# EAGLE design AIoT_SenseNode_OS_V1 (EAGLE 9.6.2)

## Sheet 1 of 4: ESP32-S3 Circuit
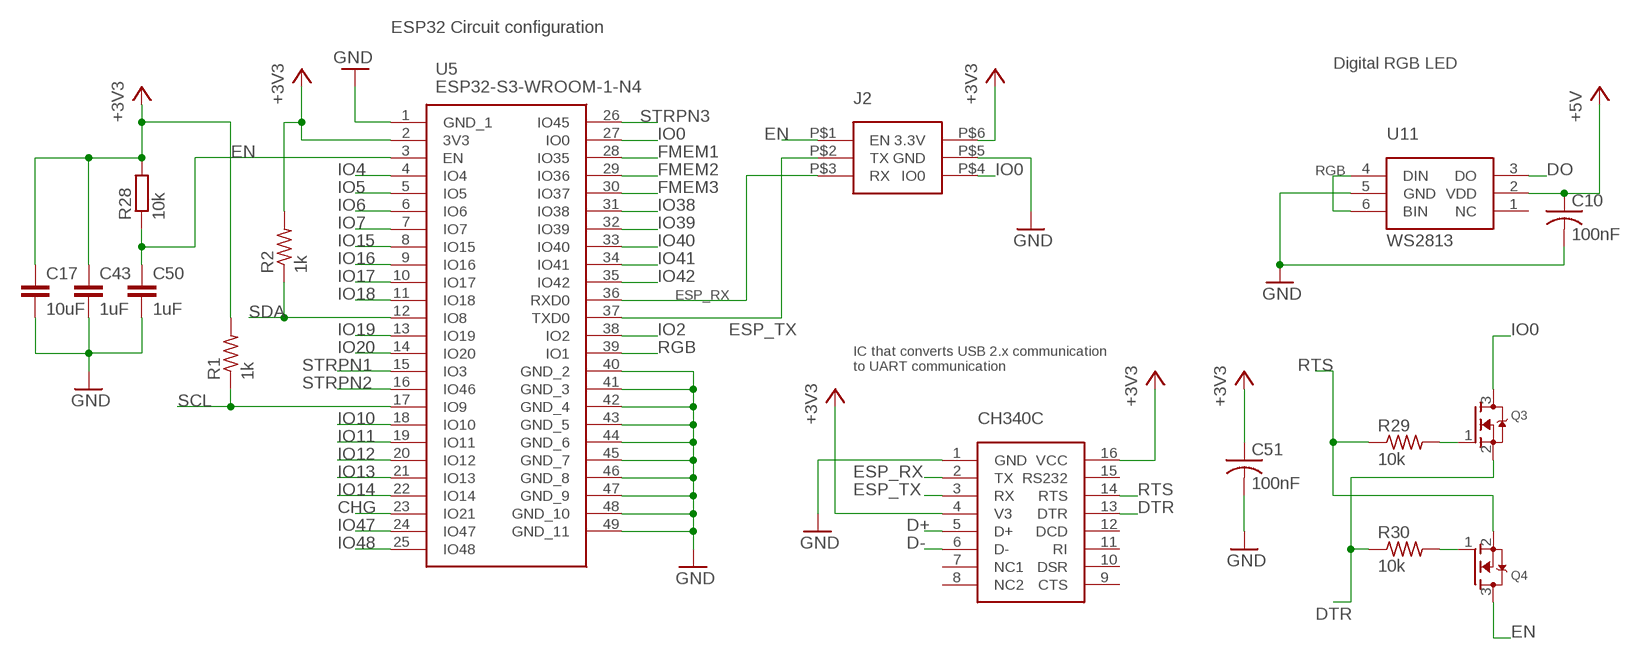
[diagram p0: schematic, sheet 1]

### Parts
C10  100nF  C-USC0603  [C0603]
C17  10uF  C-EUC0603  [C0603]
C43  1uF  C-EUC0603  [C0603]
C50  1uF  C-EUC0603  [C0603]
C51  100nF  C-USC0603  [C0603]
J2  ESP-PROG_HEADER  [2X3_1.27_HEADER]
Q3  MOSFET-NREFLOW  [SOT23-R]
Q4  MOSFET-NREFLOW  [SOT23-R]
R1  1k  R-US_R0603  [R0603]
R2  1k  R-US_R0603  [R0603]
R28  10k  R-EU_R0603  [R0603]
R29  10k  R-US_R0603  [R0603]
R30  10k  R-US_R0603  [R0603]
U5  ESP32-S3-WROOM-1-N4  [ESP32S3WROOM1N4]
U6  CH340C  [SOIC16]
U11  WS2813  [WS2813]

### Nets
+3V3: C17.1 C43.1 C51.1 J2.P$6(3.3V) R1.2 R2.2 R28.2 U5.2(3V3) U6.4(V3) U6.16(VCC) ; also sheet 2,3,4
+5V: C10.1 U11.2(VDD) ; also sheet 3
CHG: U5.23(IO21) ; also sheet 3
D+: U6.5(D+) ; also sheet 4
D-: U6.6(D-) ; also sheet 4
DO: U11.3(DO)
DTR: Q3.2(S) R30.1 U6.13(DTR)
EN: C50.1 J2.P$1(EN) Q4.3(D) R28.1 U5.3(EN) ; also sheet 4
ESP_RX: J2.P$3(RX) U5.36(RXD0) U6.2(TX)
ESP_TX: J2.P$2(TX) U5.37(TXD0) U6.3(RX)
FMEM1: U5.28(IO35)
FMEM2: U5.29(IO36)
FMEM3: U5.30(IO37)
GND: C10.2 C17.2 C43.2 C50.2 C51.2 J2.P$5(GND) U5.1(GND_1) U5.40(GND_2) U5.41(GND_3) U5.42(GND_4) U5.43(GND_5) U5.44(GND_6) U5.45(GND_7) U5.46(GND_8) U5.47(GND_9) U5.48(GND_10) U5.49(GND_11) U6.1(GND) U11.5(GND) ; also sheet 2,3,4
IO0: J2.P$4(IO0) Q3.3(D) U5.27(IO0)
IO2: U5.38(IO2) ; also sheet 4
IO4: U5.4(IO4) ; also sheet 4
IO5: U5.5(IO5) ; also sheet 4
IO6: U5.6(IO6) ; also sheet 4
IO7: U5.7(IO7) ; also sheet 4
IO10: U5.18(IO10)
IO11: U5.19(IO11) ; also sheet 4
IO12: U5.20(IO12) ; also sheet 4
IO13: U5.21(IO13) ; also sheet 4
IO14: U5.22(IO14) ; also sheet 4
IO15: U5.8(IO15) ; also sheet 4
IO16: U5.9(IO16) ; also sheet 4
IO17: U5.10(IO17) ; also sheet 4
IO18: U5.11(IO18) ; also sheet 4
IO19: U5.13(IO19) ; also sheet 4
IO20: U5.14(IO20) ; also sheet 4
IO38: U5.31(IO38) ; also sheet 4
IO39: U5.32(IO39) ; also sheet 4
IO40: U5.33(IO40) ; also sheet 4
IO41: U5.34(IO41) ; also sheet 4
IO42: U5.35(IO42) ; also sheet 4
IO47: U5.24(IO47) ; also sheet 4
IO48: U5.25(IO48) ; also sheet 4
N$3: Q4.1(G) R30.2
N$10: Q3.1(G) R29.2
RGB: U5.39(IO1) U11.4(DIN) U11.6(BIN)
RTS: Q4.2(S) R29.1 U6.14(RTS)
SCL: R1.1 U5.17(IO9) ; also sheet 2,4
SDA: R2.1 U5.12(IO8) ; also sheet 2,4
STRPN1: U5.15(IO3)
STRPN2: U5.16(IO46)
STRPN3: U5.26(IO45)
Unconnected: U6.7(NC1) U6.8(NC2) U6.9(CTS) U6.10(DSR) U6.11(RI) U6.12(DCD) U6.15(RS232) U11.1(NC)

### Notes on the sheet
- ESP32 Circuit configuration
- Digital RGB LED
- IC that converts USB 2.x communication
  to UART communication
- CH340C

## Sheet 2 of 4: ADC Circuits
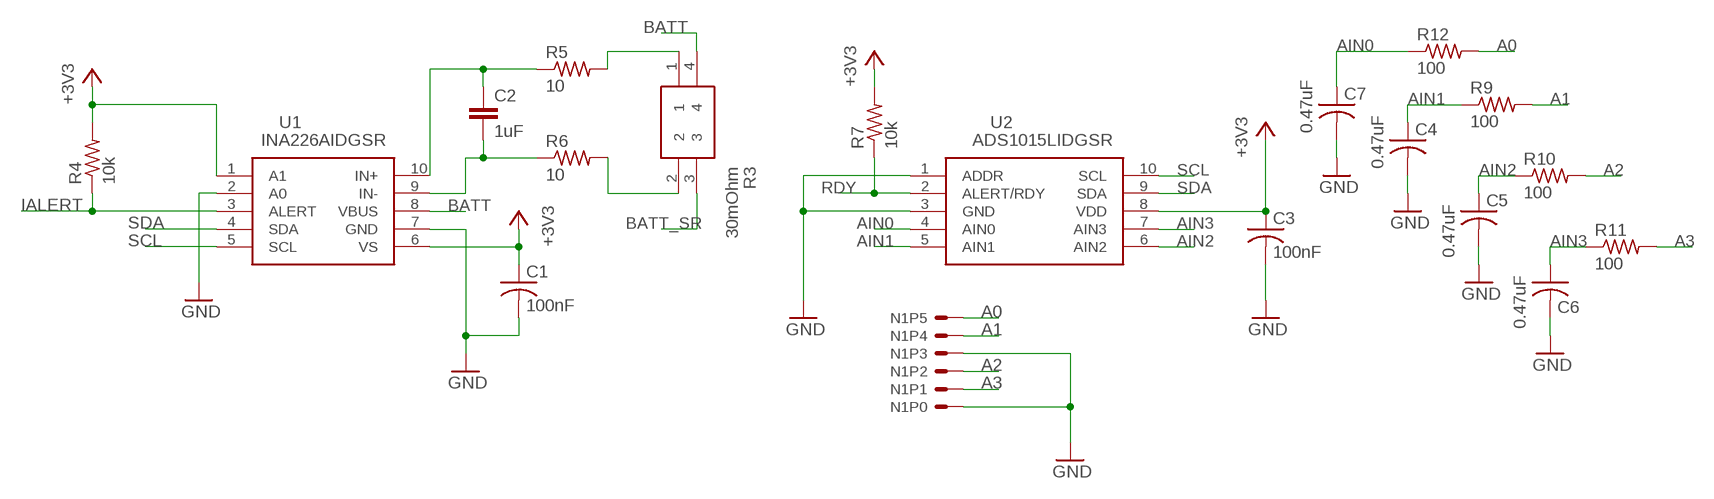
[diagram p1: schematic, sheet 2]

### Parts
C1  100nF  C-USC0603  [C0603]
C2  1uF  C-EUC0603  [C0603]
C3  100nF  C-USC0603  [C0603]
C4  0.47uF  C-USC0603  [C0603]
C5  0.47uF  C-USC0603  [C0603]
C6  0.47uF  C-USC0603  [C0603]
C7  0.47uF  C-USC0603  [C0603]
N1  6PINHEADER  [6PINHEADER]
R3  30mOhm  L4CL1206LR100DNR  [L4CL1206LR100DNR]
R4  10k  R-US_R0603  [R0603]
R5  10  R-US_R0603  [R0603]
R6  10  R-US_R0603  [R0603]
R7  10k  R-US_R0603  [R0603]
R9  100  R-US_R0603  [R0603]
R10  100  R-US_R0603  [R0603]
R11  100  R-US_R0603  [R0603]
R12  100  R-US_R0603  [R0603]
U1  INA226AIDGSR  [SOP50P490X110-10N]
U2  ADS1015LIDGSR  [SOP50P490X110-10N]

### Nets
+3V3: C1.1 C3.1 R4.2 R7.2 U1.1(A1) U1.6(VS) U2.8(VDD) ; also sheet 1,3,4
A0: N1.P5 R12.2
A1: N1.P4 R9.2
A2: N1.P2 R10.2
A3: N1.P1 R11.2
AIN0: C7.1 R12.1 U2.4(AIN0)
AIN1: C4.1 R9.1 U2.5(AIN1)
AIN2: C5.1 R10.1 U2.6(AIN2)
AIN3: C6.1 R11.1 U2.7(AIN3)
BATT: R3.4 U1.8(VBUS) ; also sheet 3,4
BATT_SR: R3.3 ; also sheet 3
GND: C1.2 C3.2 C4.2 C5.2 C6.2 C7.2 N1.P0 N1.P3 U1.2(A0) U1.7(GND) U2.1(ADDR) U2.3(GND) ; also sheet 1,3,4
IALERT: R4.1 U1.3(ALERT)
N$4: C2.1 R5.1 U1.10(IN+)
N$5: C2.2 R6.1 U1.9(IN-)
N$6: R3.1 R5.2
N$7: R3.2 R6.2
RDY: R7.1 U2.2(ALERT/RDY)
SCL: U1.5(SCL) U2.10(SCL) ; also sheet 1,4
SDA: U1.4(SDA) U2.9(SDA) ; also sheet 1,4

## Sheet 3 of 4: Power Circuits
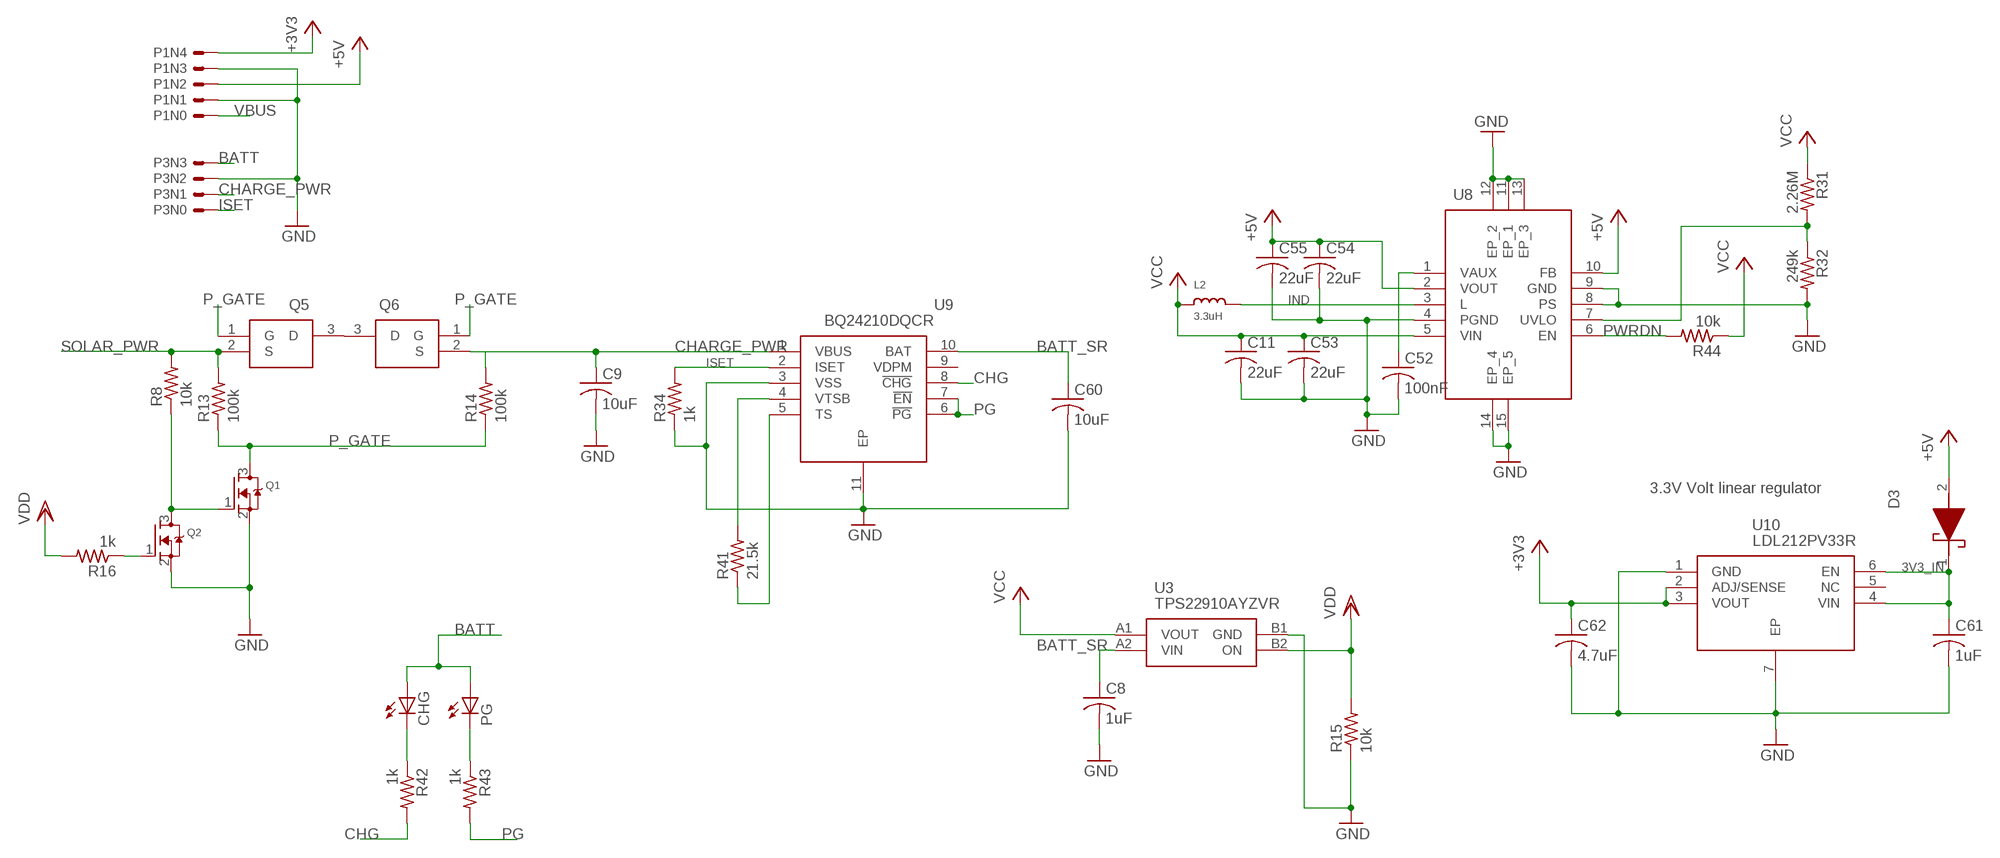
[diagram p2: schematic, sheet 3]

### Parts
C8  1uF  C-USC0603  [C0603]
C9  10uF  C-USC0603  [C0603]
C11  22uF  C-USC0603  [C0603]
C52  100nF  C-USC0603  [C0603]
C53  22uF  C-USC0603  [C0603]
C54  22uF  C-USC0603  [C0603]
C55  22uF  C-USC0603  [C0603]
C60  10uF  C-USC0603  [C0603]
C61  1uF  C-USC0603  [C0603]
C62  4.7uF  C-USC0603  [C0603]
CHG  LEDCHIPLED_0603  [CHIPLED_0603]
D3  CUS10S30,H3F  [CUZ10V]
L2  3.3uH  NRS3015T2R2MNGH  [3015_INDUCTOR]
P1  5PINHEADER  [5PINHEADER]
P3  4PINHEADER  [4PINHEADER]
PG  LEDCHIPLED_0603  [CHIPLED_0603]
Q1  MOSFET-NREFLOW  [SOT23-R]
Q2  MOSFET-NREFLOW  [SOT23-R]
Q5  SI2333CDS-T1-BE3  [SOT95P237X112-3N]
Q6  SI2333CDS-T1-BE3  [SOT95P237X112-3N]
R8  10k  R-US_R0603  [R0603]
R13  100k  R-US_R0603  [R0603]
R14  100k  R-US_R0603  [R0603]
R15  10k  R-US_R0603  [R0603]
R16  1k  R-US_R0603  [R0603]
R31  2.26M  R-US_R0603  [R0603]
R32  249k  R-US_R0603  [R0603]
R34  1k  R-US_R0603  [R0603]
R41  21.5k  R-US_R0603  [R0603]
R42  1k  R-US_R0603  [R0603]
R43  1k  R-US_R0603  [R0603]
R44  10k  R-US_R0603  [R0603]
U3  TPS22910AYZVR  [BGA4C50P2X2_89X89X50]
U8  TPS61202DRCT  [TPS61202DRCT]
U9  BQ24210DQCR  [SON50P200X300X80-11N]
U10  LDL212PV33R  [SON50P200X200X80-7N]

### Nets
3V3_IN: C61.1 D3.1(K) U10.4(VIN) U10.6(EN)
+3V3: C62.1 P1.N4 U10.2(ADJ/SENSE) U10.3(VOUT) ; also sheet 1,2,4
+5V: C54.1 C55.1 D3.2(A) P1.N2 U8.2(VOUT) U8.10(FB) ; also sheet 1
BATT: CHG.A P3.N3 PG.A ; also sheet 2,4
BATT_SR: C8.1 C60.1 U3.A2(VIN) U9.10(BAT) ; also sheet 2
CHARGE_PWR: C9.1 P3.N1 Q6.2(S) R14.2 U9.1(VBUS) ; also sheet 4
CHG: R42.2 U9.8(!CHG) ; also sheet 1
GND: C8.2 C9.2 C11.2 C52.2 C53.2 C54.2 C55.2 C60.2 C61.2 C62.2 P1.N1 P1.N3 P3.N2 Q1.2(S) Q2.2(S) R15.1 R32.2 R34.1 U3.B1(GND) U8.4(PGND) U8.8(PS) U8.9(GND) U8.11(EP_1) U8.12(EP_2) U8.13(EP_3) U8.14(EP_4) U8.15(EP_5) U9.3(VSS) U9.11(EP) U10.1(GND) U10.7(EP) ; also sheet 1,2,4
IND: L2.P$2 U8.3(L)
ISET: P3.N0 R34.2 U9.2(ISET)
N$8: Q1.1(G) Q2.3(D) R8.1
N$9: Q2.1(G) R16.1
N$11: Q5.3(D) Q6.3(D)
N$12: R31.2 R32.1 U8.7(UVLO)
N$13: C52.1 U8.1(VAUX)
N$19: R41.2 U9.4(VTSB)
N$20: R41.1 U9.5(TS)
N$21: CHG.C R42.1
N$22: PG.C R43.1
P_GATE: Q1.3(D) Q5.1(G) Q6.1(G) R13.1 R14.1
PG: R43.2 U9.6(!PG) U9.7(!EN)
PWRDN: R44.2 U8.6(EN) ; also sheet 4
SOLAR_PWR: Q5.2(S) R8.2 R13.2 ; also sheet 4
VBUS: P1.N0 ; also sheet 4
VCC: C11.1 C53.1 L2.P$1 R31.1 R44.1 U3.A1(VOUT) U8.5(VIN) ; also sheet 4
VDD: R15.2 R16.2 U3.B2(ON) ; also sheet 4
Unconnected: U9.9(VDPM) U10.5(NC)

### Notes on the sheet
- 3.3uH
- 3.3V Volt linear regulator

## Sheet 4 of 4: Connectors
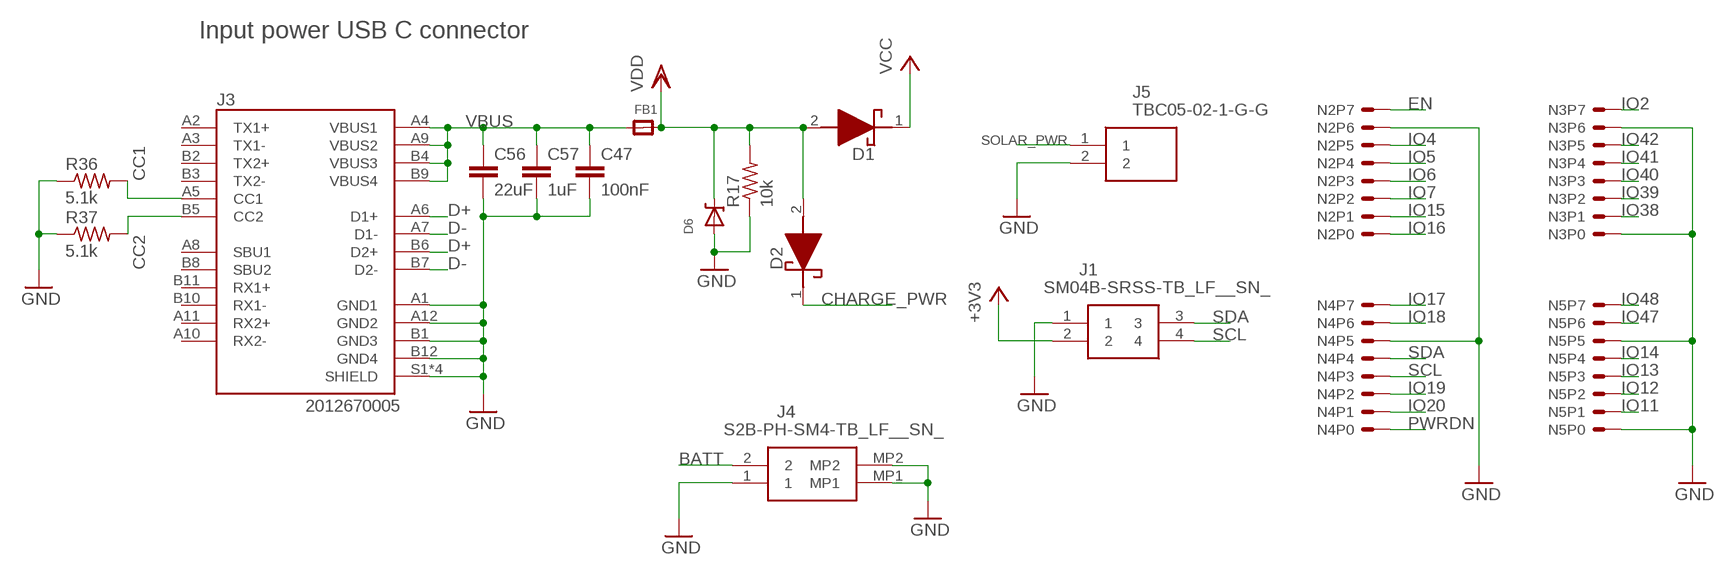
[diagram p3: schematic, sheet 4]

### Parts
C47  100nF  C-EUC0603  [C0603]
C56  22uF  C-EUC0603  [C0603]
C57  1uF  C-EUC0603  [C0603]
D1  CUS10S30,H3F  [CUZ10V]
D2  CUS10S30,H3F  [CUZ10V]
D6  DDZ5V6ASF  [DDZ5V6ASF]
FB1  FERRITE_0603  [_0603]
J1  SM04B-SRSS-TB_LF__SN_  [SM04B-SRSS-TB(LFSN)]
J3  2012670005  [MOLEX_2012670005]
J4  S2B-PH-SM4-TB_LF__SN_  [S2BPHSM4TBLFSN]
J5  TBC05-02-1-G-G  [TBC05021GG]
N2  8PINHEADER  [8PINHEADER]
N3  8PINHEADER  [8PINHEADER]
N4  8PINHEADER  [8PINHEADER]
N5  8PINHEADER  [8PINHEADER]
R17  10k  R-US_R0603  [R0603]
R36  5.1k  R-US_R0603  [R0603]
R37  5.1k  R-US_R0603  [R0603]

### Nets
+3V3: J1.2 ; also sheet 1,2,3
BATT: J4.2 ; also sheet 2,3
CC1: J3.A5(CC1) R36.2
CC2: J3.B5(CC2) R37.2
CHARGE_PWR: D2.1(K) ; also sheet 3
D+: J3.A6(D1+) J3.B6(D2+) ; also sheet 1
D-: J3.A7(D1-) J3.B7(D2-) ; also sheet 1
EN: N2.P7 ; also sheet 1
GND: C47.2 C56.2 C57.2 D6.P$1(A) J1.1 J3.A1(GND1) J3.A12(GND2) J3.B1(GND3) J3.B12(GND4) J3.S1(SHIELD) J3.S2(SHIELD) J3.S3(SHIELD) J3.S4(SHIELD) J4.1 J4.MP1 J4.MP2 J5.2 N2.P6 N3.P0 N3.P6 N4.P5 N5.P0 N5.P5 R17.1 R36.1 R37.1 ; also sheet 1,2,3
IO2: N3.P7 ; also sheet 1
IO4: N2.P5 ; also sheet 1
IO5: N2.P4 ; also sheet 1
IO6: N2.P3 ; also sheet 1
IO7: N2.P2 ; also sheet 1
IO11: N5.P1 ; also sheet 1
IO12: N5.P2 ; also sheet 1
IO13: N5.P3 ; also sheet 1
IO14: N5.P4 ; also sheet 1
IO15: N2.P1 ; also sheet 1
IO16: N2.P0 ; also sheet 1
IO17: N4.P7 ; also sheet 1
IO18: N4.P6 ; also sheet 1
IO19: N4.P2 ; also sheet 1
IO20: N4.P1 ; also sheet 1
IO38: N3.P1 ; also sheet 1
IO39: N3.P2 ; also sheet 1
IO40: N3.P3 ; also sheet 1
IO41: N3.P4 ; also sheet 1
IO42: N3.P5 ; also sheet 1
IO47: N5.P6 ; also sheet 1
IO48: N5.P7 ; also sheet 1
PWRDN: N4.P0 ; also sheet 3
SCL: J1.4 N4.P3 ; also sheet 1,2
SDA: J1.3 N4.P4 ; also sheet 1,2
SOLAR_PWR: J5.1 ; also sheet 3
VBUS: C47.1 C56.1 C57.1 FB1.1 J3.A4(VBUS1) J3.A9(VBUS2) J3.B4(VBUS3) J3.B9(VBUS4) ; also sheet 3
VCC: D1.1(K) ; also sheet 3
VDD: D1.2(A) D2.2(A) D6.P$2(C) FB1.2 R17.2 ; also sheet 3
Unconnected: J3.A2(TX1+) J3.A3(TX1-) J3.A8(SBU1) J3.A10(RX2-) J3.A11(RX2+) J3.B2(TX2+) J3.B3(TX2-) J3.B8(SBU2) J3.B10(RX1-) J3.B11(RX1+)

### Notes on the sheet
- Input power USB C connector

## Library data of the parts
C1 C3-C11 C51-C55 C60-C62 = rcl:C-US: CAPACITOR, American symbol; SPICEPREFIX: C
C2 C17 C43 C47 C50 C56 C57 = rcl:C-EU: CAPACITOR, European symbol; SPICEPREFIX: C
CHG PG = adafruit:LED: LED
D1-D3 = SamacSys_Parts:CUS10S30,H3F: Schottky Diodes & Rectifiers Single High-speed switching; DESCRIPTION: Schottky Diodes & Rectifiers Single High-speed switching; HEIGHT: 1.1mm; MANUFACTURER_NAME: Toshiba; MANUFACTURER_PART_NUMBER: CUS10S30,H3F; MOUSER_PART_NUMBER: 757-CUS10S30H3F; MOUSER_PRICE-STOCK: https://www.mouser.co.uk/ProductDetail/Toshiba/CUS10S30H3F?qs=cW4DzVrAanO4Xm6ySrHr7g%3D%3D
D6 = ForceTronics:DDZ5V6ASF: DDZ5V6ASF 5.42 Zener Diode
FB1 = microbuilder:FERRITE: Ferrite Bead
J1 = SamacSys_Parts:SM04B-SRSS-TB_LF__SN_: JST (JAPAN SOLDERLESS TERMINALS) - SM04B-SRSS-TB(LF)(SN) - CONNECTOR, HEADER, SMT, R/A, 1MM, 4WAY Source: Datasheet; DESCRIPTION: JST (JAPAN SOLDERLESS TERMINALS) - SM04B-SRSS-TB(LF)(SN) - CONNECTOR, HEADER, SMT, R/A, 1MM, 4WAY; HEIGHT: mm; MANUFACTURER_NAME: JST (JAPAN SOLDERLESS TERMINALS); MANUFACTURER_PART_NUMBER: SM04B-SRSS-TB(LF)(SN); MOUSER_PART_NUMBER: 306-SM04BSRSSTBLFSN; MOUSER_PRICE-STOCK: https://www.mouser.co.uk/ProductDetail/JST-Commercial/SM04B-SRSS-TBLFSN?qs=cdbOS8ANM9B3FdyA6cNU2A%3D%3D
J2 = ForceTronics:ESP-PROG_HEADER: 2x3 programming header for the ESP32 with 1.27mm spacing
J3 = 2012670005:2012670005: USB-C (USB TYPE-C) USB 3.1 (USB 3.1 Gen 2, Superspeed+) Receptacle Connector 24 Position Surface Mount, Right Angle; Through Hole Check availability; AVAILABILITY: In Stock; DESCRIPTION: USB-C (USB TYPE-C) USB 3.2 Gen 2 (USB 3.1 Gen 2, Superspeed + (USB 3.1)) Receptacle Connector 24 Position Surface Mount, Right Angle; Through Hole; MF: Molex; MP: 2012670005; PACKAGE: None; PRICE: None; PURCHASE-URL: https://pricing.snapeda.com/search/part/2012670005/?ref=eda
J4 = SamacSys_Parts:S2B-PH-SM4-TB_LF__SN_: Conn Shrouded Header (4 Sides) HDR 2 POS 2mm Solder RA Side Entry SMD T/R Source: Datasheet; DESCRIPTION: Conn Shrouded Header (4 Sides) HDR 2 POS 2mm Solder RA Side Entry SMD T/R; HEIGHT: 6.6mm; MANUFACTURER_NAME: JST (JAPAN SOLDERLESS TERMINALS); MANUFACTURER_PART_NUMBER: S2B-PH-SM4-TB(LF)(SN); MOUSER_PART_NUMBER: N/A; MOUSER_PRICE-STOCK: https://www.mouser.co.uk/ProductDetail/JST-Commercial/S2B-PH-SM4-TBLFSN?qs=QpmGXVUTftEA9IU90i0xlg%3D%3D
J5 = SamacSys_Parts:TBC05-02-1-G-G: Fixed Terminal Blocks 2w, 2.54mm Pitch Term-Block, Side Entry, TH, Rising Clamp; DESCRIPTION: Fixed Terminal Blocks 2w, 2.54mm Pitch Term-Block, Side Entry, TH, Rising Clamp; HEIGHT: 8.8mm; MANUFACTURER_NAME: GCT (GLOBAL CONNECTOR TECHNOLOGY); MANUFACTURER_PART_NUMBER: TBC05-02-1-G-G
L2 = ForceTronics:NRS3015T2R2MNGH: NRS3015T2R2MNGH Power Inductors - SMD 3015 2.2uH 69.6mOhms +/-20%Tol 1480mA
N1 = ForceTronics:6PINHEADER
N2-N5 = ForceTronics:8PINHEADER: 8 pin header with 2.54mm spacing
P1 = ForceTronics:5PINHEADER
P3 = ForceTronics:4PINHEADER
Q1-Q4 = microbuilder:MOSFET-N: N-Channel Mosfet LEGEND VDS: Voltage Drain-Source ID: Drain Current RDS(ON): Drain-Source On-State Resistance VGS(TH): Gate-Source Threshold Voltage CISS: Drain-Source Input Capacitance SOT-23 Name VDS ID RDS(ON) VGS(TH) CISS Order Number 2N7002E 60V 260mA 2.5 Ohm 2.5V @ 250uA 26.7pF @ 25V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
Q5 Q6 = SamacSys_Parts:SI2333CDS-T1-BE3: MOSFET P-CHANNEL 12-V (D-S) Source: Datasheet; DESCRIPTION: MOSFET P-CHANNEL 12-V (D-S); HEIGHT: 1.12mm; MANUFACTURER_NAME: Vishay; MANUFACTURER_PART_NUMBER: SI2333CDS-T1-BE3; MOUSER_PART_NUMBER: 78-SI2333CDS-T1-BE3; MOUSER_PRICE-STOCK: https://www.mouser.co.uk/ProductDetail/Vishay-Siliconix/SI2333CDS-T1-BE3?qs=CiayqK2gdcLKByimzq%252BdDA%3D%3D
R1 R2 R4-R17 R29-R32 R34 R36 R37 R41-R44 = rcl:R-US_: RESISTOR, American symbol; SPICEPREFIX: R
R3 = SamacSys_Parts:L4CL1206LR100DNR: Current Sense Resistors - SMD 4T L4CL1206 0.5W 30ppm 100 mOhm +/-0.5% ` Source: Datasheet; DESCRIPTION: Current Sense Resistors - SMD 4T L4CL1206 0.5W 30ppm 100 mOhm +/-0.5% `; HEIGHT: 0.8mm; MANUFACTURER_NAME: LITTELFUSE; MANUFACTURER_PART_NUMBER: L4CL1206LR100DNR; MOUSER_PART_NUMBER: 576-L4CL1206LR100DNR; MOUSER_PRICE-STOCK: https://www.mouser.co.uk/ProductDetail/Littelfuse/L4CL1206LR100DNR?qs=Jm2GQyTW%2Fbi3sBABnfXVtg%3D%3D
R28 = rcl:R-EU_: RESISTOR, European symbol; SPICEPREFIX: R
U1 = SamacSys_Parts:INA226AIDGSR: 36-V, Bi-Directional, Ultra-High Accuracy, Low-/High-Side, I2C Out Current/Power Monitor w/ Alert Source: Datasheet; DESCRIPTION: 36-V, Bi-Directional, Ultra-High Accuracy, Low-/High-Side, I2C Out Current/Power Monitor w/ Alert; HEIGHT: 1.1mm; MANUFACTURER_NAME: Texas Instruments; MANUFACTURER_PART_NUMBER: INA226AIDGSR; MOUSER_PART_NUMBER: 595-INA226AIDGSR; MOUSER_PRICE-STOCK: https://www.mouser.co.uk/ProductDetail/Texas-Instruments/INA226AIDGSR?qs=tQG3bEuiOZD4quG3egR36g%3D%3D
U2 = SamacSys_Parts:ADS1015LIDGSR: Analog to Digital Converters - ADC 12-bit 3.3-kSPS fou r-channel delta-sigm Source: Datasheet; DESCRIPTION: Analog to Digital Converters - ADC 12-bit 3.3-kSPS fou r-channel delta-sigm; HEIGHT: 1.1mm; MANUFACTURER_NAME: Texas Instruments; MANUFACTURER_PART_NUMBER: ADS1015LIDGSR; MOUSER_PART_NUMBER: 595-ADS1015LIDGSR; MOUSER_PRICE-STOCK: https://www.mouser.co.uk/ProductDetail/Texas-Instruments/ADS1015LIDGSR?qs=2wMNvWM5ZX4Z9D3W5OO6Eg%3D%3D
U3 = SamacSys_Parts:TPS22910AYZVR: 5.5V, 2A, 61m active-low load switch with reverse current protection Source: Datasheet; DESCRIPTION: 5.5V, 2A, 61m active-low load switch with reverse current protection; HEIGHT: 0.5mm; MANUFACTURER_NAME: Texas Instruments; MANUFACTURER_PART_NUMBER: TPS22910AYZVR; MOUSER_PART_NUMBER: 595-TPS22910AYZVR; MOUSER_PRICE-STOCK: https://www.mouser.co.uk/ProductDetail/Texas-Instruments/TPS22910AYZVR?qs=luhu8ESwuKxMmMNtGQ7xTg%3D%3D
U5 = ESP32-S3-WROOM-1-N4:ESP32-S3-WROOM-1-N4: WiFi Modules - 802.11 [Engineering Samples] SMD Module, ESP32-S3, 4 MB SPI Flash, PCB Antenna Source: Datasheet; DESCRIPTION: WiFi Modules - 802.11 [Engineering Samples] SMD Module, ESP32-S3, 4 MB SPI Flash, PCB Antenna; HEIGHT: 3.25mm; MANUFACTURER_NAME: Espressif Systems; MANUFACTURER_PART_NUMBER: ESP32-S3-WROOM-1-N4; MOUSER_PART_NUMBER: 356-ESP32-S3WROOM1N4; MOUSER_PRICE-STOCK: https://www.mouser.co.uk/ProductDetail/Espressif-Systems/ESP32-S3-WROOM-1-N4?qs=Li%252BoUPsLEnsO%2FkiJOUK0FQ%3D%3D
U6 = ForceTronics:CH340C: CH340C IC that converts USB to UART
U8 = TPS61202DRCT:TPS61202DRCT: Boost Switching Regulator IC Positive Fixed 5V 1 Output 1.2A (Switch) 10-VFDFN Exposed Pad Source: Datasheet; DESCRIPTION: Boost Switching Regulator IC Positive Fixed 5V 1 Output 1.2A (Switch) 10-VFDFN Exposed Pad; HEIGHT: 1mm; MANUFACTURER_NAME: Texas Instruments; MANUFACTURER_PART_NUMBER: TPS61202DRCT; MOUSER_PART_NUMBER: 595-TPS61202DRCT; MOUSER_PRICE-STOCK: https://www.mouser.co.uk/ProductDetail/Texas-Instruments/TPS61202DRCT?qs=KS%252B%252BetD%2FUt8d6PinTZv4Zg%3D%3D
U9 = SamacSys_Parts:BQ24210DQCR: Battery Management 800mA,Sgl-Inp,Li-Ion Solar Batt Charger Source: Datasheet; DESCRIPTION: Battery Management 800mA,Sgl-Inp,Li-Ion Solar Batt Charger; HEIGHT: 0.8mm; MANUFACTURER_NAME: Texas Instruments; MANUFACTURER_PART_NUMBER: BQ24210DQCR; MOUSER_PART_NUMBER: 595-BQ24210DQCR; MOUSER_PRICE-STOCK: https://www.mouser.co.uk/ProductDetail/Texas-Instruments/BQ24210DQCR?qs=O1HRStiETCh94UK1Y6ZDYg%3D%3D
U10 = SamacSys_Parts:LDL212PV33R: LDO Voltage Regulators VFDFPN 6 2x2x0.75 PITCH 0.5 Source: Datasheet; DESCRIPTION: LDO Voltage Regulators VFDFPN 6 2x2x0.75 PITCH 0.5; HEIGHT: 0.8mm; MANUFACTURER_NAME: STMicroelectronics; MANUFACTURER_PART_NUMBER: LDL212PV33R; MOUSER_PART_NUMBER: 511-LDL212PV33R; MOUSER_PRICE-STOCK: https://www.mouser.co.uk/ProductDetail/STMicroelectronics/LDL212PV33R?qs=5aG0NVq1C4xm%252BbuBme%252BLZw%3D%3D
U11 = ForceTronics:WS2813: WS2813 Intelligent control integrated LED light source Device

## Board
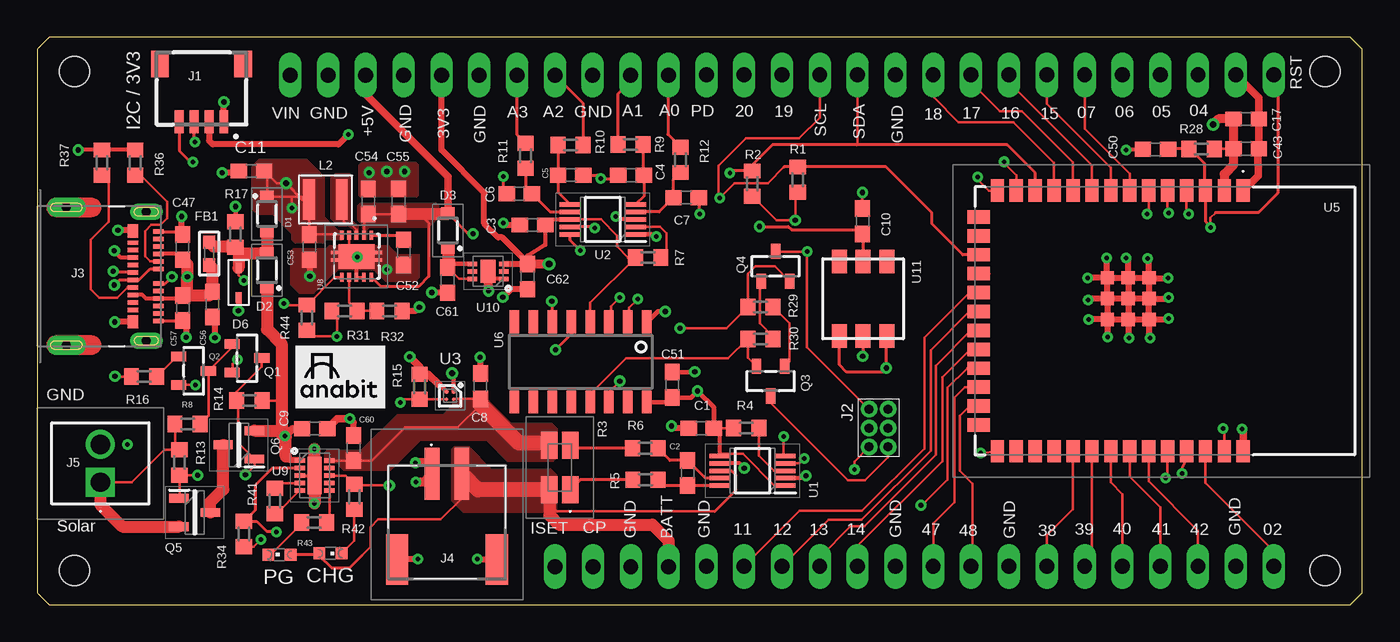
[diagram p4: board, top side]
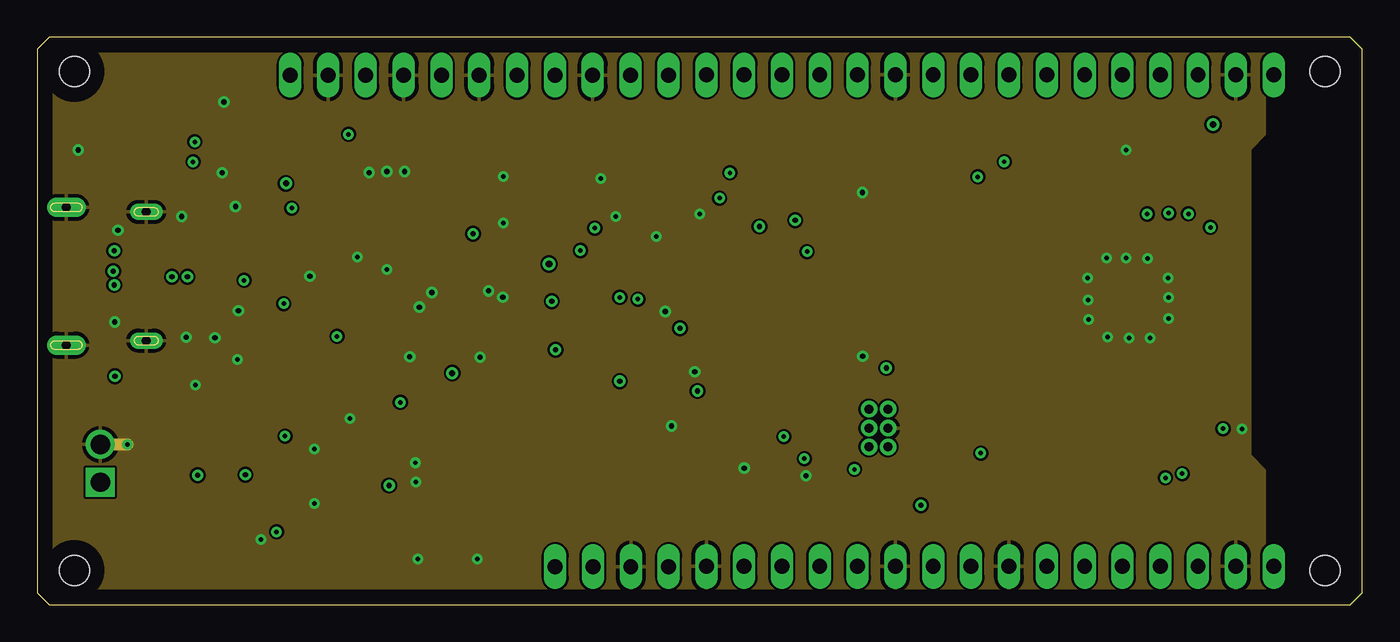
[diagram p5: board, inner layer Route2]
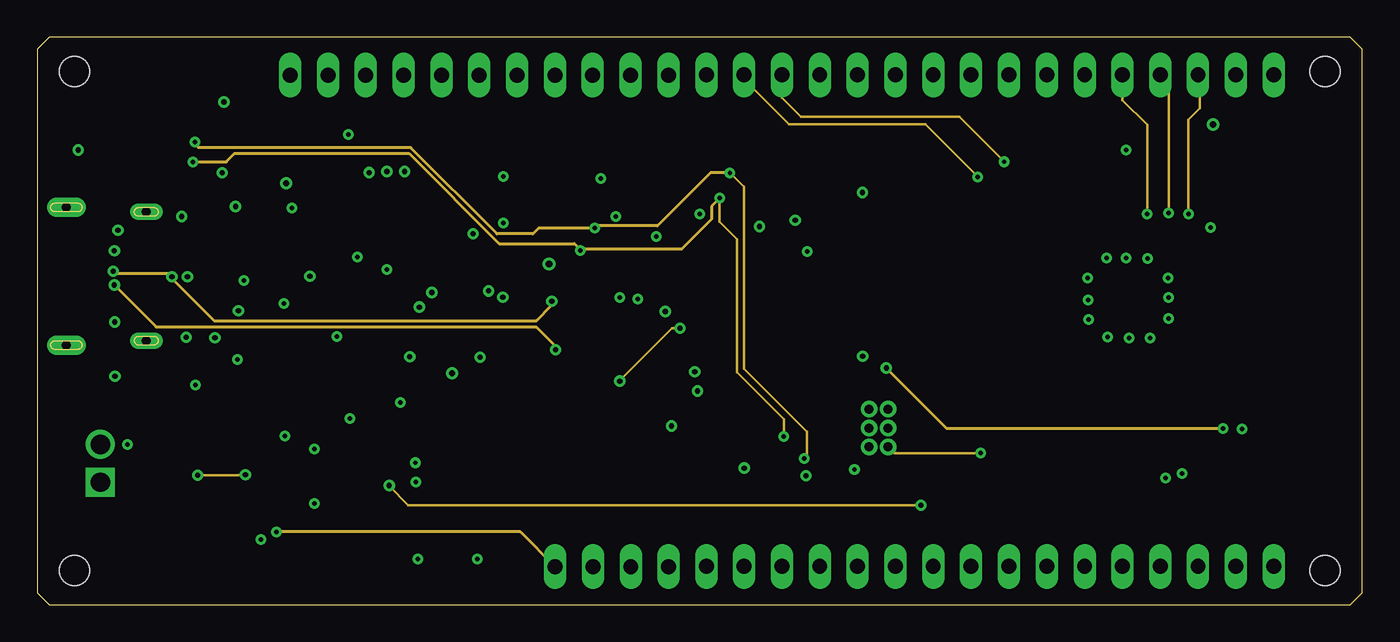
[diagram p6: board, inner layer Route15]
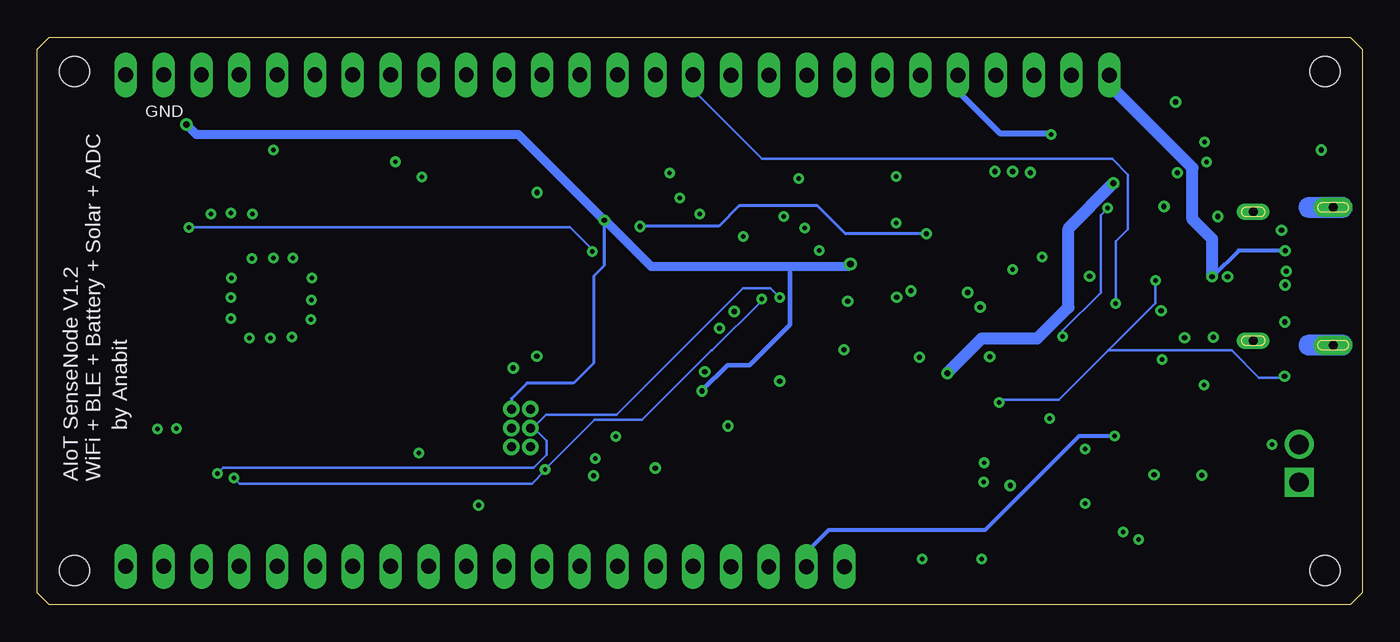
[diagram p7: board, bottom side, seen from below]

Size 89 x 38.1 mm. Coordinates in mm from the lower left corner, seen from the top.
Outline: 0.8,0 88.2,0 89,0.8 89,37.3 88.2,38.1 0.8,38.1 0,37.3 0,0.8 0.8,0
Copper layers (1+2*15+16): Top 0.035mm / dielectric 0.5mm / Route2 0.035mm / dielectric 0.5mm / Route15 0.035mm / dielectric 0.5mm / Bottom 0.035mm
Design rules "default *": minimum track width 6mil, minimum drill 0.3mm, track to track 6mil, track to pad 6mil, pad to pad 6mil, via to via 6mil, smd to smd 6mil, copper to edge 40mil, drill to drill 6mil, minimum pad ring 10mil, minimum via ring 8mil, stop-mask expansion 4mil, vias tented up to drill 0mil, thermal gap 10mil
Holes 2 mm at 2.5,2.3 2.5,35.8 86.5,2.3 86.5,35.8

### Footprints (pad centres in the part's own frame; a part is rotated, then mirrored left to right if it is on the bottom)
C0603 = smd 1.1 x 1: 1 -0.85,0; 2 0.85,0
CHIPLED_0603 = smd 0.8 x 0.8: A 0,-0.75; C 0,0.75
CUZ10V = smd 0.9 x 0.8: 1 0,-1.15; 2 0,1.15
DDZ5V6ASF = smd 0.71 x 0.41: P$1 0,0; P$2 1.99,0
_0603 = smd 0.9 x 0.8: 1 -0.762,0; 2 0.762,0
SM04B-SRSS-TB(LFSN) = smd 0.6 x 1.55: 1 1.5,4.661; 2 2.5,4.661; 3 3.5,4.661; 4 4.5,4.661 | smd 1.2 x 1.8: 5 0.2,0.786; 6 5.8,0.786
2X3_1.27_HEADER = drill 0.6 pad 0.9: P$1 0,0; P$2 1.27,0; P$3 2.54,0; P$4 2.54,1.27; P$5 1.27,1.27; P$6 0,1.27
MOLEX_2012670005 = smd 0.3 x 0.7: A1 -3,0.81; A2 -2.5,0.81; A3 -2,0.81; A4 -1.5,0.81; A5 -1,0.81; A6 -0.5,0.81; A7 0.5,0.81; A8 1,0.81; A9 1.5,0.81; A10 2,0.81; A11 2.5,0.81; A12 3,0.81; B2 2.25,-0.89; B3 1.75,-0.89; B4 1.25,-0.89; B5 0.75,-0.89; B6 0.25,-0.89; B7 -0.25,-0.89; B8 -0.75,-0.89; B9 -1.25,-0.89; B10 -1.75,-0.89; B11 -2.25,-0.89 | smd 0.9 x 0.7: B1 3.05,-0.89; B12 -3.05,-0.89 | drill 0.6 pad 1.1 long: S1 -4.32,0; S2 4.32,0 | drill 0.6 pad 1.3 long: S3 -4.62,-5.36; S4 4.62,-5.36
S2BPHSM4TBLFSN = smd 1 x 3.5: 1 1,-3.25; 2 -1,-3.25 | smd 1.5 x 3.4: MP1 3.35,2.5; MP2 -3.35,2.5
TBC05021GG = drill 1.3 pad 1.95 square: 1 0,0 | drill 1.3 pad 1.95: 2 2.54,0
3015_INDUCTOR = smd 0.8 x 2.7: P$1 0,0; P$2 2.2,0
6PINHEADER = drill 1 long: P0 1.27,-1.778; P1 3.81,-1.778; P2 6.35,-1.778; P3 8.89,-1.778; P4 11.43,-1.778; P5 13.97,-1.778
8PINHEADER = drill 1 long: P0 1.27,-3.81; P1 3.81,-3.81; P2 6.35,-3.81; P3 8.89,-3.81; P4 11.43,-3.81; P5 13.97,-3.81; P6 16.51,-3.81; P7 19.05,-3.81
5PINHEADER = drill 1 long: N0 -5.08,0; N1 -2.54,0; N2 0,0; N3 2.54,0; N4 5.08,0
4PINHEADER = drill 1 long: N0 -3.81,0; N1 -1.27,0; N2 1.27,0; N3 3.81,0
SOT23-R = smd 0.635 x 1.016: 1 -0.95,-1; 2 0.95,-1; 3 0,1
SOT95P237X112-3N = smd 1.3 x 0.6: 1 -1.05,0.95; 2 -1.05,-0.95; 3 1.05,0
R0603 = smd 1 x 1.1: 1 -0.85,0; 2 0.85,0
L4CL1206LR100DNR = smd 1.8 x 1.1: 1 -1.5,-0.7; 2 1.5,-0.7; 3 1.5,0.7; 4 -1.5,0.7
SOP50P490X110-10N = smd 1.4 x 0.3: 1 -2.2,1; 2 -2.2,0.5; 3 -2.2,0; 4 -2.2,-0.5; 5 -2.2,-1; 6 2.2,-1; 7 2.2,-0.5; 8 2.2,0; 9 2.2,0.5; 10 2.2,1
BGA4C50P2X2_89X89X50 = smd 0.221 x 0.221: A1 -0.25,0.25; A2 0.25,0.25; B1 -0.25,-0.25; B2 0.25,-0.25
ESP32S3WROOM1N4 = smd 1.5 x 0.9: 1 -8.75,5.26; 2 -8.75,3.99; 3 -8.75,2.72; 4 -8.75,1.45; 5 -8.75,0.18; 6 -8.75,-1.09; 7 -8.75,-2.36; 8 -8.75,-3.63; 9 -8.75,-4.9; 10 -8.75,-6.17; 11 -8.75,-7.44; 12 -8.75,-8.71; 13 -8.75,-9.98; 14 -8.75,-11.25; 27 8.75,-11.25; 28 8.75,-9.98; 29 8.75,-8.71; 30 8.75,-7.44; 31 8.75,-6.17; 32 8.75,-4.9; 33 8.75,-3.63; 34 8.75,-2.36; 35 8.75,-1.09; 36 8.75,0.18; 37 8.75,1.45; 38 8.75,2.72; 39 8.75,3.99; 40 8.75,5.26 | smd 0.9 x 1.5: 15 -6.985,-12.5; 16 -5.715,-12.5; 17 -4.445,-12.5; 18 -3.175,-12.5; 19 -1.905,-12.5; 20 -0.635,-12.5; 21 0.635,-12.5; 22 1.905,-12.5; 23 3.175,-12.5; 24 4.445,-12.5; 25 5.715,-12.5; 26 6.985,-12.5 | smd 0.9 x 0.9: 41 -1.5,-2.46; 42 -0.1,-2.46; 43 -0.1,-1.06; 44 -1.5,-1.06; 45 -2.9,-1.06; 46 -2.9,-2.46; 47 -2.9,-3.86; 48 -1.5,-3.86; 49 -0.1,-3.86
SOIC16 = smd 0.635 x 1.524: 1 -4.445,-2.695; 2 -3.175,-2.695; 3 -1.905,-2.695; 4 -0.635,-2.695; 5 0.635,-2.695; 6 1.905,-2.695; 7 3.175,-2.695; 8 4.445,-2.695; 9 4.445,2.695; 10 3.175,2.695; 11 1.905,2.695; 12 0.635,2.695; 13 -0.635,2.695; 14 -1.905,2.695; 15 -3.175,2.695; 16 -4.445,2.695
TPS61202DRCT = smd 0.6 x 0.24: 1 -1.4,1; 2 -1.4,0.5; 3 -1.4,0; 4 -1.4,-0.5; 5 -1.4,-1; 6 1.4,-1; 7 1.4,-0.5; 8 1.4,0; 9 1.4,0.5; 10 1.4,1 | smd 1.65 x 2.4: 11 0,0 | smd 0.25 x 0.5: 12 -0.25,1.45; 13 0.25,1.45; 14 -0.25,-1.45; 15 0.25,-1.45
SON50P200X300X80-11N = smd 0.7 x 0.3: 1 -1,1; 2 -1,0.5; 3 -1,0; 4 -1,-0.5; 5 -1,-1; 6 1,-1; 7 1,-0.5; 8 1,0; 9 1,0.5; 10 1,1 | smd 0.94 x 2.5: 11 0,0
SON50P200X200X80-7N = smd 0.65 x 0.3: 1 -1.05,0.5; 2 -1.05,0; 3 -1.05,-0.5; 4 1.05,-0.5; 5 1.05,0; 6 1.05,0.5 | smd 1.02 x 1.55: 7 0,0
WS2813 = smd 1.6 x 1: 1 5.2,1.1; 2 5.2,2.7; 3 5.2,4.3; 4 0.2,4.3; 5 0.2,2.7; 6 0.2,1.1

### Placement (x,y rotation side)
C1  44.6,11.85 180 top
C2  43.69,8.84 90 top
C3  33.27,25.49 180 top
C4  39.89,28.84 180 top
C5  35.83,28.84 0 top
C6  32.38,27.6 180 top
C7  43.59,27.33 0 top
C8  29.77,14.67 90 top
C9  18.64,11.82 0 top
C10  55.44,25.75 90 top
C11  14.39,29.12 180 top
C17  81.2,32.61 0 top
C43  81.2,30.61 0 top
C47  9.77,24.01 90 top
C50  75.11,30.57 180 top
C51  42.65,14.76 90 top
C52  24.61,23.65 270 top
C53  18.28,24.01 270 top
C54  22.24,27.07 90 top
C55  24.28,27.08 90 top
C56  11.77,20.16 270 top
C57  9.78,19.92 270 top
C60  21.26,10.52 90 top
C61  27.56,21.79 270 top
C62  32.93,22.03 270 top
CHG  19.7,3.44 270 top
D1  15.44,26.23 180 top
D2  15.43,22.46 0 top
D3  27.59,25.12 0 top
D6  13.53,20.63 90 top
FB1  11.55,23.57 90 top
J1  14.04,37.09 180 top
J2  55.87,13.13 270 top
J3  7.32,22.05 270 top
J4  27.52,5.53 180 top
J5  4.24,8.22 90 top
L2  18.26,27.2 0 top
N1  28.42,37.33 0 top
N2  64,39.38 0 top
N3  64,6.38 0 top
N4  43.67,39.38 0 top
N5  43.67,6.38 0 top
P1  22.07,35.56 0 top
P3  38.6,2.55 0 top
PG  16.28,3.36 90 top
Q1  14.09,16.55 270 top
Q2  10.5,15.7 270 top
Q3  49.26,15.01 180 top
Q4  49.59,22.72 0 top
Q5  10.58,6.19 0 top
Q6  13.54,10.73 180 top
R1  51.09,28.54 270 top
R2  48.03,28.27 270 top
R3  35.1,9.21 90 top
R4  47.62,11.85 180 top
R5  40.85,8.39 180 top
R6  40.84,10.5 180 top
R7  41.03,23.31 180 top
R8  10.1,12.14 180 top
R9  39.85,30.91 180 top
R10  35.82,30.87 0 top
R11  32.8,30.14 90 top
R12  43.21,29.87 90 top
R13  9.56,9.55 90 top
R14  14.25,13.7 0 top
R15  25.68,14.63 270 top
R16  7.18,15.31 180 top
R17  13.32,24.86 270 top
R28  78.2,30.6 0 top
R29  48.58,20 0 top
R30  48.58,17.85 0 top
R31  20.64,19.72 0 top
R32  23.66,19.72 0 top
R34  13.89,4.75 90 top
R36  6.58,29.68 270 top
R37  4.35,29.68 270 top
R41  15.97,6.96 90 top
R42  21.3,7.24 90 top
R43  18.6,5.51 0 top
R44  18.12,19.27 90 top
U1  48.04,8.99 180 top
U2  37.99,25.87 180 top
U3  27.73,14.03 270 top
U5  75.74,19.05 270 top
U6  36.5,16.3 180 top
U8  21.45,23.39 270 top
U9  18.63,8.67 0 top
U10  30.28,22.38 180 top
U11  58.17,17.84 90 top

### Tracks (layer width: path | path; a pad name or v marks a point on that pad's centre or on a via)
3V3_IN
  Top 0.152: C61.1 28.32,21.88 U10.6
  Top 0.305: U10.4 27.8,22.88 27.59,22.67
  Top 0.813: D3.1 27.59,22.67 C61.1
+3V3  (via drill 0.3, 0.35, 0.45)
  Top 0.152: U10.2 U10.3 | U2.8 37.86,25.87 38.95,24.78 38.95,24.05 39.69,23.31 R7.2 37.13,20.27 U6.4 | R4.2 C1.1 | C43.1 R28.2 | R2.2 49.65,25.8 v50.91,25.8 50.91,27.52 R1.2 | U1.6 45.97,10.12 47.4,10.12 49.56,7.96 50.21,7.96 U1.1
  Top 0.254: U2.8 34.57,25.87 C3.1 34.12,24.16 32.93,23.44 C62.1 33.24,22.88 | C1.1 45.84,11.46 U1.6
  Top 0.305: U6.16 42.34,13.61 C51.1 43.92,13.91 v44.35,14.35 45.45,13.25 C1.1
  Top 0.406: U10.3 C62.1 32.93,22.96 31.23,24.66 30.96,24.66 30.03,25.59 30.03,27.65 27.15,30.53 P1.N4 | v20.91,31.58 20.24,30.91 11.79,30.91 11.54,31.16 J1.2
  Top 0.61: v34.38,22.87 C62.1 | v78.97,32.24 79.34,32.61 C17.1 C43.1 80.35,29.54 79.72,28.91 U5.2
  Bottom 0.203: v50.91,25.8 50.91,22.77 51.63,22.05 51.63,16.22 52.98,14.87 56.1,14.87 57.14,13.83 J2.P$6
  Bottom 0.305: 38.45,22.71 38.45,18.79 41.16,16.08 42.65,16.08 44.37,14.36 v44.35,14.35
  Bottom 0.406: P1.N4 27.15,34.46 24.35,31.66 20.99,31.66 v20.91,31.58
  Bottom 0.61: v34.38,22.87 34.54,22.71 38.45,22.71 47.77,22.71 50.89,25.83 v50.91,25.8 56.69,31.58 78.31,31.58 v78.97,32.24
+5V  (via drill 0.35)
  Top 0.152: U8.2 21.95,25.93 C54.1 C55.1
  Top 0.2: C55.1 25.7,26.23 26.3,25.63 26.3,22.05 25.6,21.35 23.09,21.35 U8.10 | D3.2 28.99,24.87 29.28,24.87 v29.28,24.9 | v48.51,25.39 50.44,25.39 50.65,25.17 55.17,25.17 C10.1 55.47,24.87 U11.2
  Top 0.254: D3.2 27.75,26.27
  Top 0.508: D3.2 27.59,28.74 22.07,34.26 P1.N2
  Top 0.813: D3.2 27.55,26.23 C55.1
  Bottom 0.2: v29.28,24.9 34.7,24.9 36.58,26.78 41.85,26.78 43.21,25.42 48.48,25.42 v48.51,25.39
  pour Top (no thermals): 26.8,26.95 21.7,26.95 21.5,26.75 21.5,25.85 21.82,25.53 21.82,24.55 22.15,24.55 22.15,25.2 22.3,25.35 26.3,25.35 27,26.05 27,26.75
A0
  Top 0.2: R12.2 42.36,31.57 42.36,35.52 N1.P5
A1
  Top 0.2: R9.2 39,34.29 39.85,35.14 N1.P4
A2
  Top 0.2: N1.P2 36.67,33.65 R10.2
A3
  Top 0.2: N1.P1 32.2,35.52 32.2,31.59 R11.2
AIN0
  Top 0.2: U2.4 41.78,26.37 C7.1 42.74,28.55 R12.1
AIN1
  Top 0.2: R9.1 40.7,28.88 C4.1 40.74,27.42 U2.5
AIN2
  Top 0.2: R10.1 C5.1 34.98,27.68 U2.6
AIN3
  Top 0.2: R11.1 32.8,28.03 C6.1 34.46,26.37 U2.7
BATT
  Top 0.152: 21.8,3.3 22.38,3.88 22.38,5.19 22.91,5.72 27.1,5.72 28.52,7.14 J4.2 | 45.51,6.27 34.9,6.27 34.4,6.77
  Top 0.2: 21.8,3.3 20.95,2.45 19.8,2.45 18.95,3.3 CHG.A 18.87,3.36 PG.A | U1.8 46.63,8.99 46.89,8.73 46.89,7.65 45.51,6.27 | 34.5,7.68 34.4,7.68
  Top 0.61: R3.4 34.4,7.68
  Top 0.813: R3.4 34.4,6.77 34.4,6 35.02,5.38 41.32,5.38 42.41,4.29 P3.N3
  Top 1.016: R3.4 29.59,7.71 J4.2 29.14,8.16
  pour Top (no thermals): 30.5,9.1 29,10.6 28,10.6 27.8,10.4 27.8,7 28.6,6.2 34.9,6.2 34.9,8.7 34.5,9.1
BATT_SR
  Top 0.152: U9.10 C60.1 22.47,9.67 24.7,11.9 28.24,11.9 29.77,13.43 | U3.A2 28.02,13.82 C8.1
  Top 1.016: R3.3 34.27,10.84 32.36,10.84 29.77,13.43
  pour Top (no thermals): 23.7,9 20.6,9 20.3,9.3 20.3,9.5 19.3,9.5 19.3,10.2 19.5,10.4 21.8,10.4 24.2,12.8 27.3,12.8 27.9,13.4 27.9,13.8 28,13.9 30.1,13.9 31.8,12.2 34.5,12.2 34.9,11.8 34.9,9.9 34.6,9.6 31.6,9.6 30.2,11 25.7,11
CC1
  Top 0.152: J3.A5 7.58,23.05 7.24,23.39 7.24,25.08 7.66,25.5 8.29,25.5 8.72,25.93 8.72,27.05 6.94,28.83 R36.2
CC2
  Top 0.152: 6.37,21.24 J3.B5 6.07,21.3 5.38,20.61 4.16,20.61 3.6,21.17 3.6,24.49 4.81,25.7 4.81,28.37 R37.2
CHARGE_PWR  (via drill 0.3)
  Top 0.152: R14.2 16.42,13.7 16.43,13.69 | v16.64,11.32 16.43,11.53 16.43,11.62
  Top 0.203: U9.1 17.63,9.7
  Top 0.254: 16.35,11.54 16.43,11.62 16.54,11.73 16.66,11.85 | 16.7,11.26 v16.64,11.32
  Top 0.406: 17.63,9.7 16.95,9.7 16.7,9.95
  Top 0.508: v16.64,11.32 17.14,11.82 C9.1
  Top 0.61: 16.37,11.78 16.35,11.8
  Top 0.813: D2.1 15.43,18.48 16.43,17.48 16.43,13.69 16.43,11.62 | 16.7,9.95 16.7,11.26 | 16.35,11.54 16.35,11.8 | Q6.2 16.49,11.68 16.54,11.73
  Bottom 0.254: v16.64,11.32 19.02,11.32 25.34,5 35.84,5 37.33,3.51 P3.N1
CHG  (via drill 0.35)
  Top 0.152: U9.8 20.72,8.67 R42.2 21.39,8.01 v23.64,8.01 | U5.23 62.47,15.88 61.14,14.55 61.14,8.39 59.43,6.68 v59.35,6.68
  Route15 0.152: v59.35,6.68 24.92,6.68 23.62,7.98 v23.64,8.01
D+  (via drill 0.35)
  Top 0.152: J3.B6 6.41,21.78
  Top 0.203: J3.B6 6.84,21.8 7.59,22.55 J3.A6 | 6.41,21.78 5.49,21.78 v5.18,21.47 | v34.81,17.12 35.95,18.26 35.95,18.91 U6.5
  Route15 0.203: v5.18,21.47 7.99,18.66 33.51,18.66 34.81,17.36 v34.81,17.12
D-  (via drill 0.35)
  Top 0.152: J3.B7 | 5.18,22.31 v5.1,22.39
  Top 0.203: J3.A7 8.59,21.55 v9.05,22.02 | J3.B7 5.18,22.31 | v34.56,20.37 34.59,20.34 U6.6
  Route15 0.152: v9.05,22.02 9.05,21.9
  Route15 0.203: v9.05,22.02 8.83,22.24 5.25,22.24 v5.1,22.39 | 9.05,21.9 11.88,19.07 33.53,19.07 34.56,20.1 v34.56,20.37
DTR
  Top 0.152: Q3.2 47.73,16.59 R30.1 46.41,16.53 39.54,16.53 37.13,14.12 U6.13
EN  (via drill 0.3)
  Top 0.152: 79.15,26.33 78.8,25.98 78.8,25.4 v78.8,25.34 | Q4.3 v51.71,23.71 51.71,17.29 J2.P$1
  Top 0.2: U5.3 78.39,27.87 78.39,29.64 77.43,30.6 R28.1 75.99,30.6 C50.1 | 79.15,26.33 82.01,26.33 83.32,27.64 83.32,35.3 N2.P7 | U5.3 78.46,27.18 | U5.3 78.46,25.73 78.8,25.4
  Bottom 0.152: v51.71,23.71 51.65,23.77 53.22,25.34 v78.8,25.34
ESP_RX  (via drill 0.3)
  Top 0.152: v75.78,8.51 75.92,8.73 U5.36 | U6.2 39.76,19.08 39.76,19.93 v40.34,20.51 | v54.89,9.08 54.89,9.61 J2.P$3
  Bottom 0.152: v75.78,8.51 75.4,8.13 55.78,8.13 54.89,9.02 v54.89,9.08 51.57,12.4 48.37,12.4 43.7,17.07 43.67,17.07 40.28,20.46 v40.34,20.51
ESP_TX  (via drill 0.3)
  Top 0.152: U5.37 77.41,10.25 76.91,9.19 v76.91,8.8 76.94,8.77 76.94,8.62 | v39.13,20.63 38.53,20.03 38.53,19.18 38.41,19.05 U6.3
  Bottom 0.152: v76.91,8.8 76.51,9.2 55.67,9.2 54.79,10.08 54.79,11.01 55.64,11.86 55.72,11.86 | v39.13,20.63 39.76,21.26 41.59,21.26 50.1,12.75 54.83,12.75 55.72,11.86 | 55.72,11.86 J2.P$2
GND  (via drill 0.3, 0.35)
  Top 0.152: U8.4 20.95,23.89 U8.11 | R34.1 14.54,3.9 v15.02,4.38 | Q2.2 v10.62,14.76 | v13.44,16.47 13.14,16.17 13.14,15.65 Q1.2
  Top 0.2: U9.3 U9.11 | C5.2 37.61,28.84 v37.84,28.61 38.81,28.61 C4.2 | C7.2 44.44,26.3 v44.5,26.24 | C6.2 31.31,27.6 v31.31,28.76 | J3.A1 9.68,25.05 9.71,25.02 | J3.A12 9.76,19.05 C57.2 | U8.8 U8.9 | U11.5 55.47,16.7 v55.45,16.68 | C10.2 55.44,27.66 v55.42,27.68
  Top 0.254: R36.1 R37.1 v2.76,30.53 | v51.63,8.65 51.47,8.49 U1.2 | C50.2 74.23,30.54 v73.15,30.54 | U8.8 21.45,23.31 v21.5,23.36 | U10.1 30.5,21.88 30.28,21.66 | U2.3 39.05,25.87 v38.87,26.05 | v47.49,9.17 47.17,9.49 U1.7
  Top 0.305: U2.1 41.44,24.87 v41.59,24.72 | U6.1 41.01,19 41.7,19.69 v42.19,19.69 | C51.2 44.14,15.61 v44.17,15.64 | U3.B1 27,14.76 26.99,14.76 | R17.1 v13.32,26.74
  Top 0.406: C60.2 21.26,12.22 v20.99,12.49 | C3.2 31.44,25.49 v31.31,25.62 | J1.1 v12.54,33.75 | C47.2 9.71,24.92 9.71,25.02 v9.71,26.06 | J3.B12 6.39,25.14 v5.42,25.14 | C53.2 18.31,23.13 v18.31,22.05 | J3.B1 6.41,18.98 v5.21,18.98 | C57.2 10,18.85 v10,17.96 | C56.2 11.93,19.15 v11.93,17.92 | D6.P$1 13.53,19.76 v13.51,19.74 | R32.2 25.41,19.72 v25.67,19.98 | C61.2 26.53,20.94 v26.51,20.96 | C10.2 55.4,26.64 | C62.2 31.81,21.18 v31.27,20.64 | C8.2 29.77,16.59 v29.75,16.61 | C1.2 42.6,11.85 v42.6,12 | U5.49 v71.89,17.97 | U5.49 v70.62,19.15 v70.61,19.16 | U5.49 U5.42 | U5.42 73.28,17.96 v73.34,17.9 | U5.42 U5.43 | U5.43 75.92,19.15 v75.98,19.21 | U5.43 74.68,17.98 v74.74,17.92 | U5.43 U5.44 | U5.44 75.94,20.55 v76,20.61 | U5.44 U5.41 | U5.41 U5.48 | U5.48 70.66,20.55 v70.58,20.47 | U5.48 U5.47 | U5.47 71.84,21.99 v71.84,23.27 | U5.47 70.59,21.95 v70.56,21.92 | U5.46 73.28,23.14 v73.15,23.27 | U5.45 74.68,23.15 v74.58,23.25 | U5.46 U5.41 | U5.45 U5.44 | U5.45 74.71,21.92 v75.95,21.92 | U5.47 U5.46 | U5.46 U5.45 | U5.41 U5.42 | U5.48 U5.49 | v25.58,3.06 24.2,3.06 J4.MP1 | v29.55,3.06 30.84,3.06 J4.MP2 | C11.2 13.42,29 v12.43,29
  Top 0.508: J4.1 26.52,9.45 26.44,9.53 | N2.P6 82.05,34.03 C17.2 C43.2 81.98,30.54 81.98,30.25 82,28.8 U5.1 | U5.40 81,11.75 v80.94,11.81 | 26.99,14.76 26.27,15.48 R15.1 25.68,15.98 v25.02,16.64 | C9.2 20.16,12.49 v20.99,12.49
  Top 0.61: 26.44,9.53 v25.4,9.53 | v25.42,8.25 25.99,8.25 J4.1 | U10.7 30.28,21.66 30.28,21.1 v30.31,21.07
  Top 0.813: v18.62,10.44 U9.11 v18.63,6.79
  Route2 0.813: J5.2 v6.04,10.76 v6.05,10.75
  other vias: 22.3,29.01 23.48,29.08 23.48,22.5 24.68,29.08
  pour Route2: 53.5,43.05 82.5,43.05 82.5,31.55 81.5,30.55 81.5,10.05 82.5,9.05 82.5,-1.95 -3.5,-1.95 -3.5,40.05 -1.5,42.05 52.5,42.05
  pour Top (no thermals): 19.4,23.9 17.2,23.9 17,23.7 17,21.5 17.6,20.9 19.4,20.9 20,21.5 20,22.3 20.2,22.5 22.6,22.5 23.4,21.7 25.4,21.7 25.67,21.97 25.67,23.5 24.2,23.5 23.6,24.1 19.6,24.1
  pour Top (no thermals): 25.4,29.7 21.8,29.7 21.6,29.5 21.6,27.5 21.7,27.4 25.5,27.4 25.6,27.5 25.6,29.5
IALERT
  Top 0.152: R4.1 48.47,10 49.48,8.99 U1.3
IND
  Top 0.152: L2.P$2 20.57,27.09 20.57,25.76 20.78,25.55 21.08,25.55 21.45,25.18 U8.3
  pour Top (no thermals): 20,28.95 19.7,28.65 19.7,25.95 20.2,25.45 20.9,25.45 21.28,25.07 21.28,24.55 21.58,24.55 21.58,25.37 21.1,25.85 21.1,28.85 21,28.95
IO0  (via drill 0.3)
  Top 0.152: U5.27 v63.37,10.17 | Q3.3 49.26,13.56 54.47,8.35 55.6,8.35 57.14,9.89 J2.P$4
  Route15 0.152: v63.37,10.17 57.56,10.17 J2.P$4
IO2
  Top 0.152: U5.38 78.46,8.19 83.05,3.6 N3.P7
IO4  (via drill 0.3)
  Top 0.152: U5.4 77.19,26.38 v77.33,26.25
  Route15 0.152: v77.33,26.25 77.33,32.54 78.1,33.32 78.1,35.44 N2.P5
IO5  (via drill 0.3)
  Top 0.152: U5.5 75.92,26.45 75.88,26.41 v76,26.29
  Route15 0.152: v76,26.29 76,34.99 N2.P4
IO6  (via drill 0.3)
  Top 0.152: U5.6 74.65,26.42 74.55,26.32 v74.55,26.23
  Route15 0.152: v74.55,26.23 74.55,32.22 72.89,33.88 N2.P3
IO7
  Top 0.152: U5.7 73.38,28.94 70.35,31.97 N2.P2
IO10
  Top 0.152: U5.18 63.95,22.23
IO11
  Top 0.152: U5.19 62.62,20.96 59.59,17.92 59.59,10.47 55.41,6.29 51.2,6.29 N5.P1
IO12
  Top 0.152: N5.P2 53.14,5.69 55.37,5.69 60.01,10.33 60.01,17.07 62.62,19.69 U5.20
IO13
  Top 0.152: U5.21 62.73,18.41 60.35,16.04 60.35,10.05 55.56,5.26 54.63,5.26 52.56,3.19 N5.P3
IO14
  Top 0.152: U5.22 62.69,17.14 60.8,15.26 60.8,9.64 55.1,3.94 N5.P4
IO15
  Top 0.152: U5.8 72.11,29.34 67.81,33.64 N2.P1
IO16
  Top 0.152: U5.9 70.84,29.51 65.27,35.08 N2.P0
IO17
  Top 0.152: U5.10 69.57,29.71 66.15,33.13 64.67,33.13 62.72,35.08 N4.P7
IO18
  Top 0.152: U5.11 68.3,29.68 65.58,32.4 61.87,32.4 60.18,34.09 N4.P6
IO19  (via drill 0.3)
  Top 0.152: U5.13 65.76,28.84 64.91,29.69 v64.96,29.74
  Route15 0.152: v64.96,29.74 61.93,32.77 51.29,32.77 50.02,34.04 N4.P2
IO20  (via drill 0.3)
  Top 0.152: U5.14 63.92,27.8 63.18,28.54 v63.18,28.72
  Route15 0.152: v63.18,28.72 59.65,32.25 50.5,32.25 47.48,35.27 N4.P1
IO38
  Top 0.152: U5.31 69.57,6.42 67.81,4.66 N3.P1
IO39
  Top 0.152: U5.32 70.84,3.06 N3.P2
IO40
  Top 0.152: U5.33 72.11,8.21 72.89,7.43 N3.P3
IO41
  Top 0.152: U5.34 73.38,8.59 75.43,6.54 N3.P4
IO42
  Top 0.152: U5.35 74.65,8.3 77.97,4.98 N3.P5
IO47
  Top 0.152: U5.24 62.3,14.61 61.6,13.91 61.6,6.88 60.18,5.46 N5.P6
IO48
  Top 0.152: U5.25 62.62,13.34 61.96,12.67 61.96,8.98 62.81,8.13 62.81,2.66 N5.P7
ISET  (via drill 0.3)
  Top 0.203: U9.2 15.79,9.17 14.64,8.02 14.64,6.35 R34.2 14.73,5.6 15.43,4.9 v16.06,4.9 v16.07,4.89
  Route15 0.203: v16.07,4.89 32.45,4.89 P3.N0
N$3
  Top 0.152: R30.2 49.43,18 48.54,18.89 48.54,21.62 Q4.1
N$4
  Top 0.2: U1.10 C2.1
  Top 0.203: R5.1 42.1,7.99 C2.1
N$5
  Top 0.2: U1.9 44.89,8.49 C2.2
  Top 0.203: C2.2 42.5,9.69 R6.1
N$6
  Top 0.203: R5.2 36.48,8.39 R3.1
N$7
  Top 0.203: R6.2 36.01,10.5 R3.2
N$8
  Top 0.152: Q1.1 13.09,17.29 Q2.3 11.5,12.69 R8.1
N$9
  Top 0.152: R16.1 9.37,16.65 Q2.1
N$10
  Top 0.152: Q3.1 50.53,16.33 50.53,18.9 R29.2
N$11
  Top 0.813: Q5.3 11.63,6.89 12.49,7.75 Q6.3
N$12
  Top 0.152: U8.7 20.95,20.26 R31.2 R32.1
N$13
  Top 0.2: U8.1 24.32,24.79 C52.1
N$19
  Top 0.152: U9.4 16.33,8.17 R41.2
N$20
  Top 0.152: U9.5 16.07,6.11 R41.1
N$21
  Top 0.152: R42.1 21.3,4.29 CHG.C
N$22
  Top 0.152: R43.1 17.75,5.43 15.68,3.36 PG.C
P_GATE  (via drill 0.35)
  Top 0.152: Q1.3 15.09,15.98 13.4,14.29 13.4,13.81 | 13.4,13.81 R14.1 | 13.4,13.81 13.51,13.7 13.51,10.86 Q6.1 14.59,9.32 v13.99,8.72 | v10.78,8.69 v10.77,8.7 R13.1 9.56,7.17 Q5.1
  Route15 0.152: v13.99,8.72 13.96,8.69 v10.78,8.69
PG
  Top 0.152: U9.7 U9.6 19.63,5.69 R43.2
PWRDN  (via drill 0.3)
  Top 0.152: U8.6 19.98,21.98 R44.2 16.62,20.12 16.54,20.2 v16.56,20.22
  Bottom 0.152: v16.56,20.22 16.56,24.39 15.73,25.22 15.73,28.88 16.79,29.94 40.32,29.94 44.94,34.56 N4.P0
RDY
  Top 0.152: U2.2 41.83,25.37 42.27,24.93 42.27,23.7 R7.1
RGB  (via drill 0.3, 0.35)
  Top 0.152: U5.39 79.73,11.74 v79.65,11.82
  Top 0.2: U11.6 57.03,18 v57.03,15.89 56.76,15.62 54.36,15.62 53.87,16.11 U11.4
  Route15 0.2: v79.65,11.82 61.09,11.82 v57.03,15.88 v57.03,15.89
RTS  (via drill 0.35)
  Top 0.152: Q4.2 49.54,22.72 48.24,22.72 47.73,22.21 R29.1 46.29,18.56 v43.18,18.56 | v39.13,15.01 38.41,14.29 U6.14
  Route15 0.152: v43.18,18.56 42.62,18.56 39.1,15.04 v39.13,15.01
SCL  (via drill 0.3)
  Top 0.152: 50.16,29.39 49.07,28.3 46.84,28.3 v45.84,27.3 45.76,27.38 45.76,29.48 47.59,31.31 51.17,31.31 52.56,32.7 N4.P3 | v50.15,11.29 50.13,11.27 50.13,10.1 U1.5
  Top 0.2: U5.17 62.17,23.5 60.08,25.59 60.08,26.32 57.01,29.39 R1.1 50.16,29.39 | v36.48,23.78 35.79,24.47 U2.10 | J1.4 9.54,30.49 10.38,29.65 v10.46,29.73
  Route15 0.152: v45.84,27.3 45.84,25.72 47.01,24.55 47.01,15.59 50.15,12.45 v50.15,11.29
  Route15 0.2: v45.84,27.3 45.29,26.75 45.29,25.89 43.28,23.88 36.46,23.88 | v36.48,23.78 36.48,23.75 36.59,23.75 36.46,23.88 | v10.46,29.73 12.7,29.73 13.26,30.3 24.97,30.3 31.02,24.25 36.09,24.25 36.46,23.88
SDA  (via drill 0.3)
  Top 0.152: v51.52,9.81 51.2,9.49 U1.4 | N4.P4 55.1,30.95 55.03,30.88
  Top 0.2: U5.12 67.03,29 65.15,30.88 55.03,30.88 49.38,30.88 48.03,29.53 R2.1 46.7,29.12 46.57,28.99 v46.53,28.99 | v37.45,25.29 37.37,25.37 U2.9 | v10.58,31.08 10.54,31.08 J1.3
  Route15 0.152: v46.53,28.99 47.48,28.05 47.48,15.84 51.7,11.61 51.7,9.81 v51.52,9.81
  Route15 0.2: v46.53,28.99 45.21,28.99 41.65,25.43 37.49,25.43 37.45,25.39 v37.45,25.29 33.68,25.29 33.29,24.9 30.87,24.9 25.08,30.69 10.84,30.69 10.55,30.98 10.55,31.14 10.56,31.14 10.58,31.12 v10.58,31.08
SOLAR_PWR
  Top 0.152: J5.1 6.36,8.22 8.54,10.4 R13.2 9.25,10.71 R8.2
  Top 0.813: J5.1 4.24,6.72 5.72,5.24 Q5.2
VBUS  (via drill 0.35)
  Top 0.254: C47.1 9.38,23.55 J3.A4 | C57.1 9.56,20.55 J3.A9 7.31,20.55 7.06,20.8 J3.B4 | J3.B9 5.61,23.3 5.18,23.73 v5.18,23.77
  Top 0.61: C47.1 10.09,22.85 | C57.1 10.09,21.07
  Top 0.813: 10.09,22.85 v10.09,22.03 10.09,21.07 | C57.1 11.53,20.77 C56.1 11.77,22.59 FB1.1
  Bottom 0.254: v5.18,23.77 8.3,23.77 10.06,22 v10.09,22.03
  Bottom 0.813: v10.09,22.03 10.09,24.55 11.41,25.87 11.41,29.33 16.99,34.91 P1.N0
VCC  (via drill 0.3, 0.4)
  Top 0.152: 17.04,27.38 D1.1 15.44,28.92 C11.1 16.07,28.29 v16.71,28.29 | U8.5 20.38,24.86 C53.1 18.26,24.88 L2.P$1 18.07,27.39 17.03,27.39 17.04,27.38 | 17.04,27.38 17.1,27.32 v17.1,26.63 | R31.1 20.14,19.37 v20.14,18.02 18.46,18.02 18.12,18.36 R44.1
  Top 0.2: v16.71,28.29 17.8,27.2 L2.P$1
  Top 0.305: v27.87,15.55 27.98,15.44 U3.A1
  Bottom 0.152: v17.1,26.63 17.57,26.16 17.57,20.95 20.14,18.38 v20.14,18.02
  Bottom 0.813: v27.87,15.55 v27.87,15.56 25.55,17.88 21.83,17.88 19.74,19.97 19.74,25.25 v16.71,28.28 v16.71,28.29
  pour Top (no thermals): 18.1,29.9 14.9,29.9 14.4,29.4 14.4,26.6 14.8,26.2 15.8,26.2 17.1,24.9 17.1,24.5 17.3,24.3 19.2,24.3 19.4,24.5 20.5,24.5 20.6,24.6 20.6,25.1 20.2,25.1 19.3,26 19.3,28.7
VDD  (via drill 0.3, 0.35)
  Top 0.152: 24.42,13.62 v24.39,13.59 24.58,13.78 R15.2 U3.B2 | v13.88,21.78 13.53,22.13 D6.P$2 | v5.22,15.33 5.24,15.31 R16.2
  Top 0.813: D1.2 D2.2 13.72,23.61 R17.2 | FB1.2 11.84,24.04 13.29,24.04 R17.2 | R17.2 13.53,23.8 D6.P$2
  Bottom 0.152: 17.06,17.08 20.39,13.75 24.23,13.75 v24.39,13.59 | 17.06,17.08 13.88,20.25 v13.88,21.78 | 17.06,17.08 8.78,17.08 6.95,15.25 5.22,15.25 v5.22,15.33

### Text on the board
tNames: RST | +5V | GND | 3V3 | GND | PD | 20 | 19 | SCL | SDA | GND | VIN | GND | A3 | A2 | GND | A1 | A0 | 18 | 17 | 16 | 15 | 07 | 06 | 05 | 04 | I2C / 3V3 | GND | GND | GND | 11 | 12 | 13 | 14 | 47 | 48 | 02 | Solar | ISET | CP | GND | BATT | GND | 38 | 39 | 40 | 41 | 42 | GND
bNames: GND | by Anabit | AIoT SenseNode V1.2 / WiFi + BLE + Battery + Solar + ADC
